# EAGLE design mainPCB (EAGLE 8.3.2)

## Sheet 1 of 2: RPi/ADC
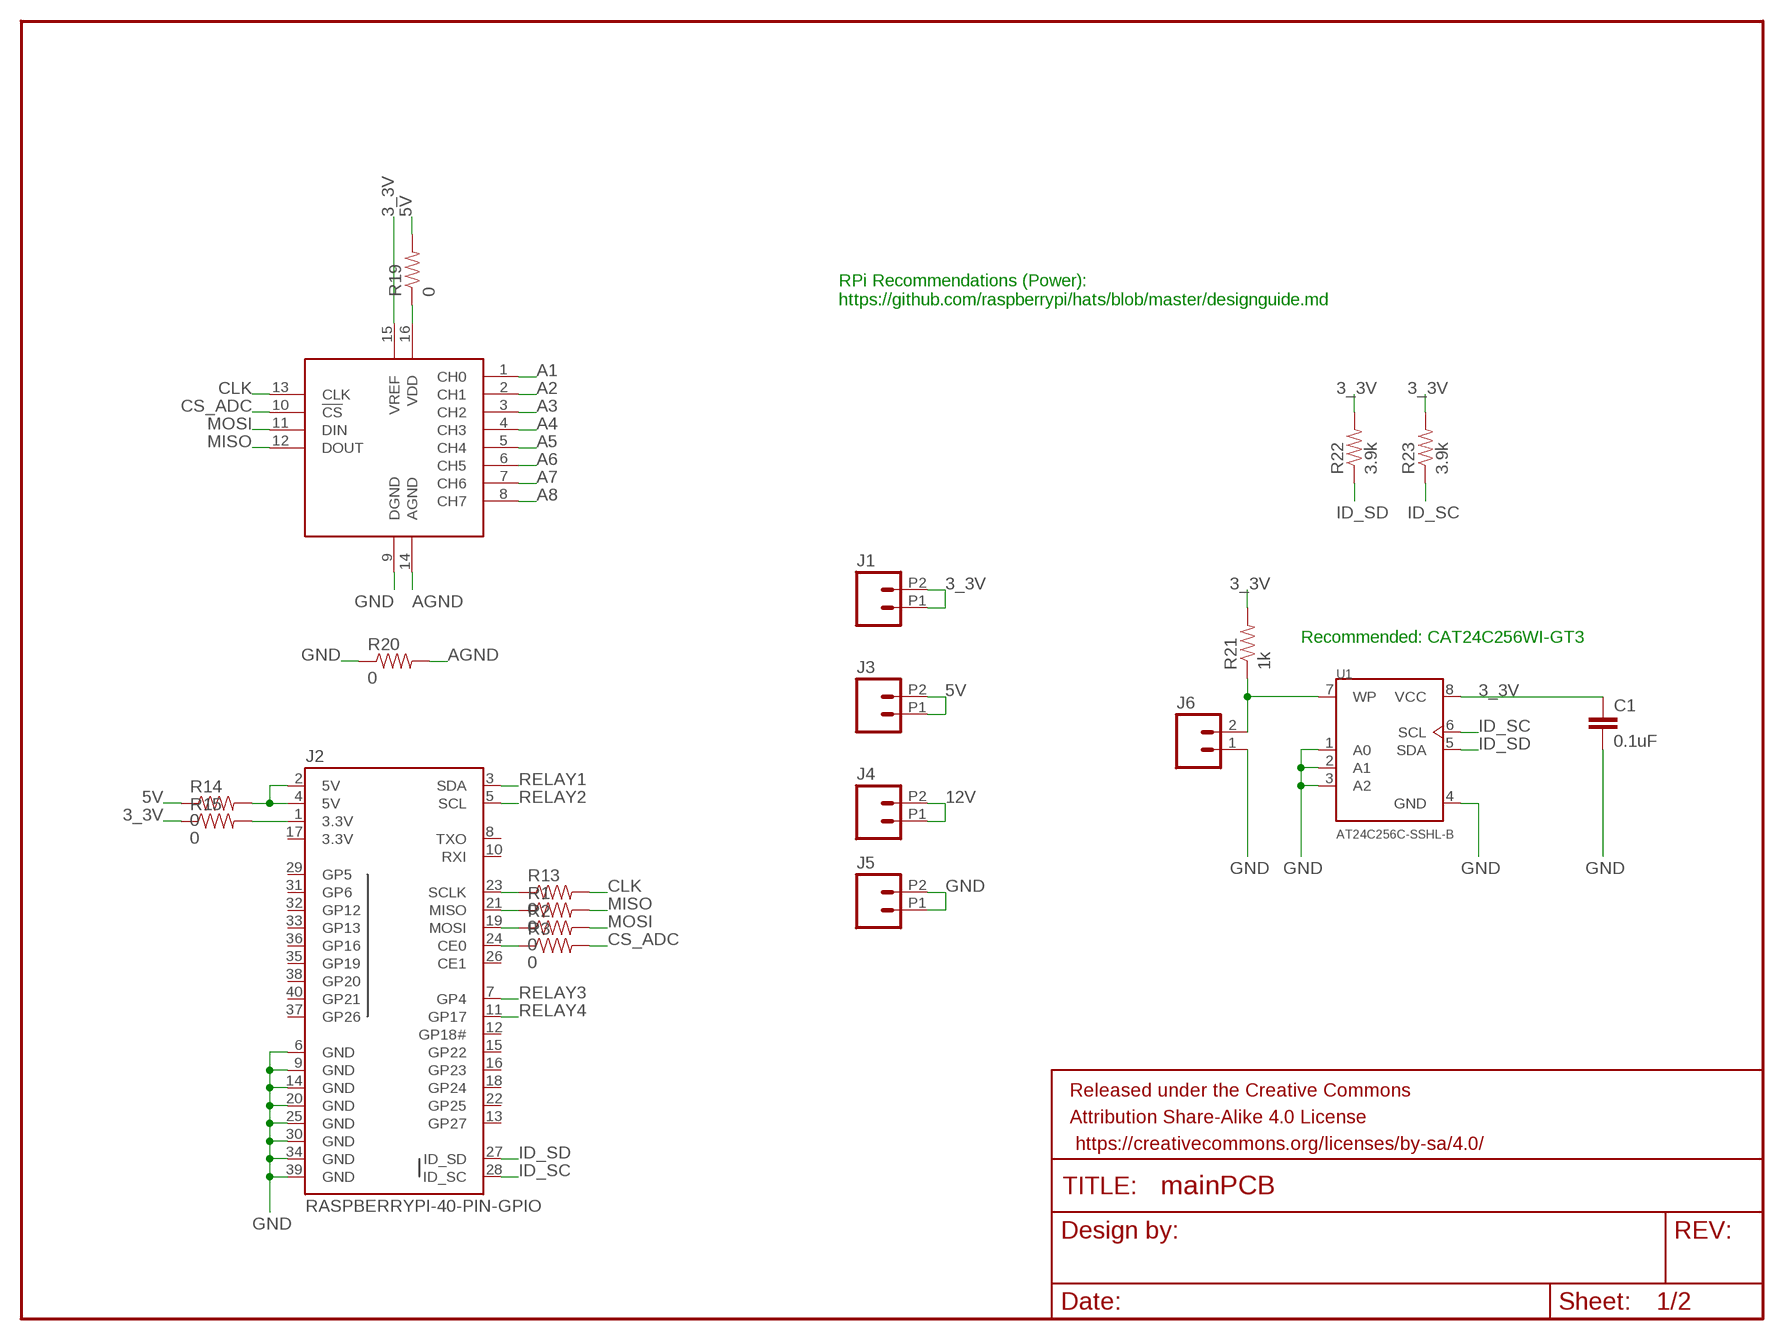
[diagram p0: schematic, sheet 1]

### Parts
C1  0.1uF  0.1UF-25V(+80/-20%)(0603)  [0603-CAP]
FRAME2  FRAME-LETTERNO_PACKAGE  [DUMMY]
J1  M022.54MM_SCREWTERM  [1X02_2.54_SCREWTERM]
J2  RASPBERRYPI-40-PIN-GPIO  [2X20-SHROUDED]
J3  M022.54MM_SCREWTERM  [1X02_2.54_SCREWTERM]
J4  M022.54MM_SCREWTERM  [1X02_2.54_SCREWTERM]
J5  M022.54MM_SCREWTERM  [1X02_2.54_SCREWTERM]
J6  M02PTH  [1X02]
R1  0  RESISTOR0603-RES  [0603-RES]
R2  0  RESISTOR0603-RES  [0603-RES]
R3  0  RESISTOR0603-RES  [0603-RES]
R13  0  RESISTOR0603-RES  [0603-RES]
R14  0  RESISTOR0603-RES  [0603-RES]
R15  0  RESISTOR0603-RES  [0603-RES]
R19  0  RESISTOR0603-RES  [0603-RES]
R20  0  RESISTOR0603-RES  [0603-RES]
R21  1k  RESISTOR0603-RES  [0603-RES]
R22  3.9k  RESISTOR0603-RES  [0603-RES]
R23  3.9k  RESISTOR0603-RES  [0603-RES]
U1  AT24C256C-SSHL-B  [SOIC127P600X175-8N]
U$1  MCP3208I/SL  [SO-16DW]

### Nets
3_3V: C1.1 J1.P1 J1.P2 R15.1 R21.2 R22.2 R23.2 U1.8(VCC) U$1.15(VREF)
5V: J3.P1 J3.P2 R14.1 R19.2 ; also sheet 2
12V: J4.P1 J4.P2 ; also sheet 2
A1: U$1.1(CH0) ; also sheet 2
A2: U$1.2(CH1) ; also sheet 2
A3: U$1.3(CH2) ; also sheet 2
A4: U$1.4(CH3) ; also sheet 2
A5: U$1.5(CH4)
A6: U$1.6(CH5)
A7: U$1.7(CH6)
A8: U$1.8(CH7)
AGND: R20.2 U$1.14(AGND)
CLK: R13.2 U$1.13(CLK)
CS_ADC: R3.2 U$1.10(!CS)
GND: C1.2 J2.6(GND) J2.9(GND) J2.14(GND) J2.20(GND) J2.25(GND) J2.30(GND) J2.34(GND) J2.39(GND) J5.P1 J5.P2 J6.1 R20.1 U1.1(A0) U1.2(A1) U1.3(A2) U1.4(GND) U$1.9(DGND) ; also sheet 2
ID_SC: J2.28(ID_SC) R23.1 U1.6(SCL)
ID_SD: J2.27(ID_SD) R22.1 U1.5(SDA)
MISO: R1.2 U$1.12(DOUT)
MOSI: R2.2 U$1.11(DIN)
N$17: J2.2(5V) J2.4(5V) R14.2
N$18: J2.1(3.3V) R15.2
N$19: J2.23(SCLK) R13.1
N$20: J2.21(MISO) R1.1
N$25: J2.19(MOSI) R2.1
N$26: J2.24(CE0) R3.1
N$27: R19.1 U$1.16(VDD)
RELAY1: J2.3(SDA) ; also sheet 2
RELAY2: J2.5(SCL) ; also sheet 2
RELAY3: J2.7(GP4) ; also sheet 2
RELAY4: J2.11(GP17) ; also sheet 2
WP: J6.2 R21.1 U1.7(WP)
Unconnected: J2.8(TXO) J2.10(RXI) J2.12(GP18#) J2.13(GP27) J2.15(GP22) J2.16(GP23) J2.18(GP24) J2.22(GP25) J2.26(CE1) J2.29(GP5) J2.31(GP6) J2.32(GP12) J2.33(GP13) J2.35(GP19) J2.36(GP16) J2.37(GP26) J2.38(GP20) J2.40(GP21)

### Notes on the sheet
- RPi Recommendations (Power):
  https://github.com/raspberrypi/hats/blob/master/designguide.md
- Recommended: CAT24C256WI-GT3

## Sheet 2 of 2: Relays 1-2
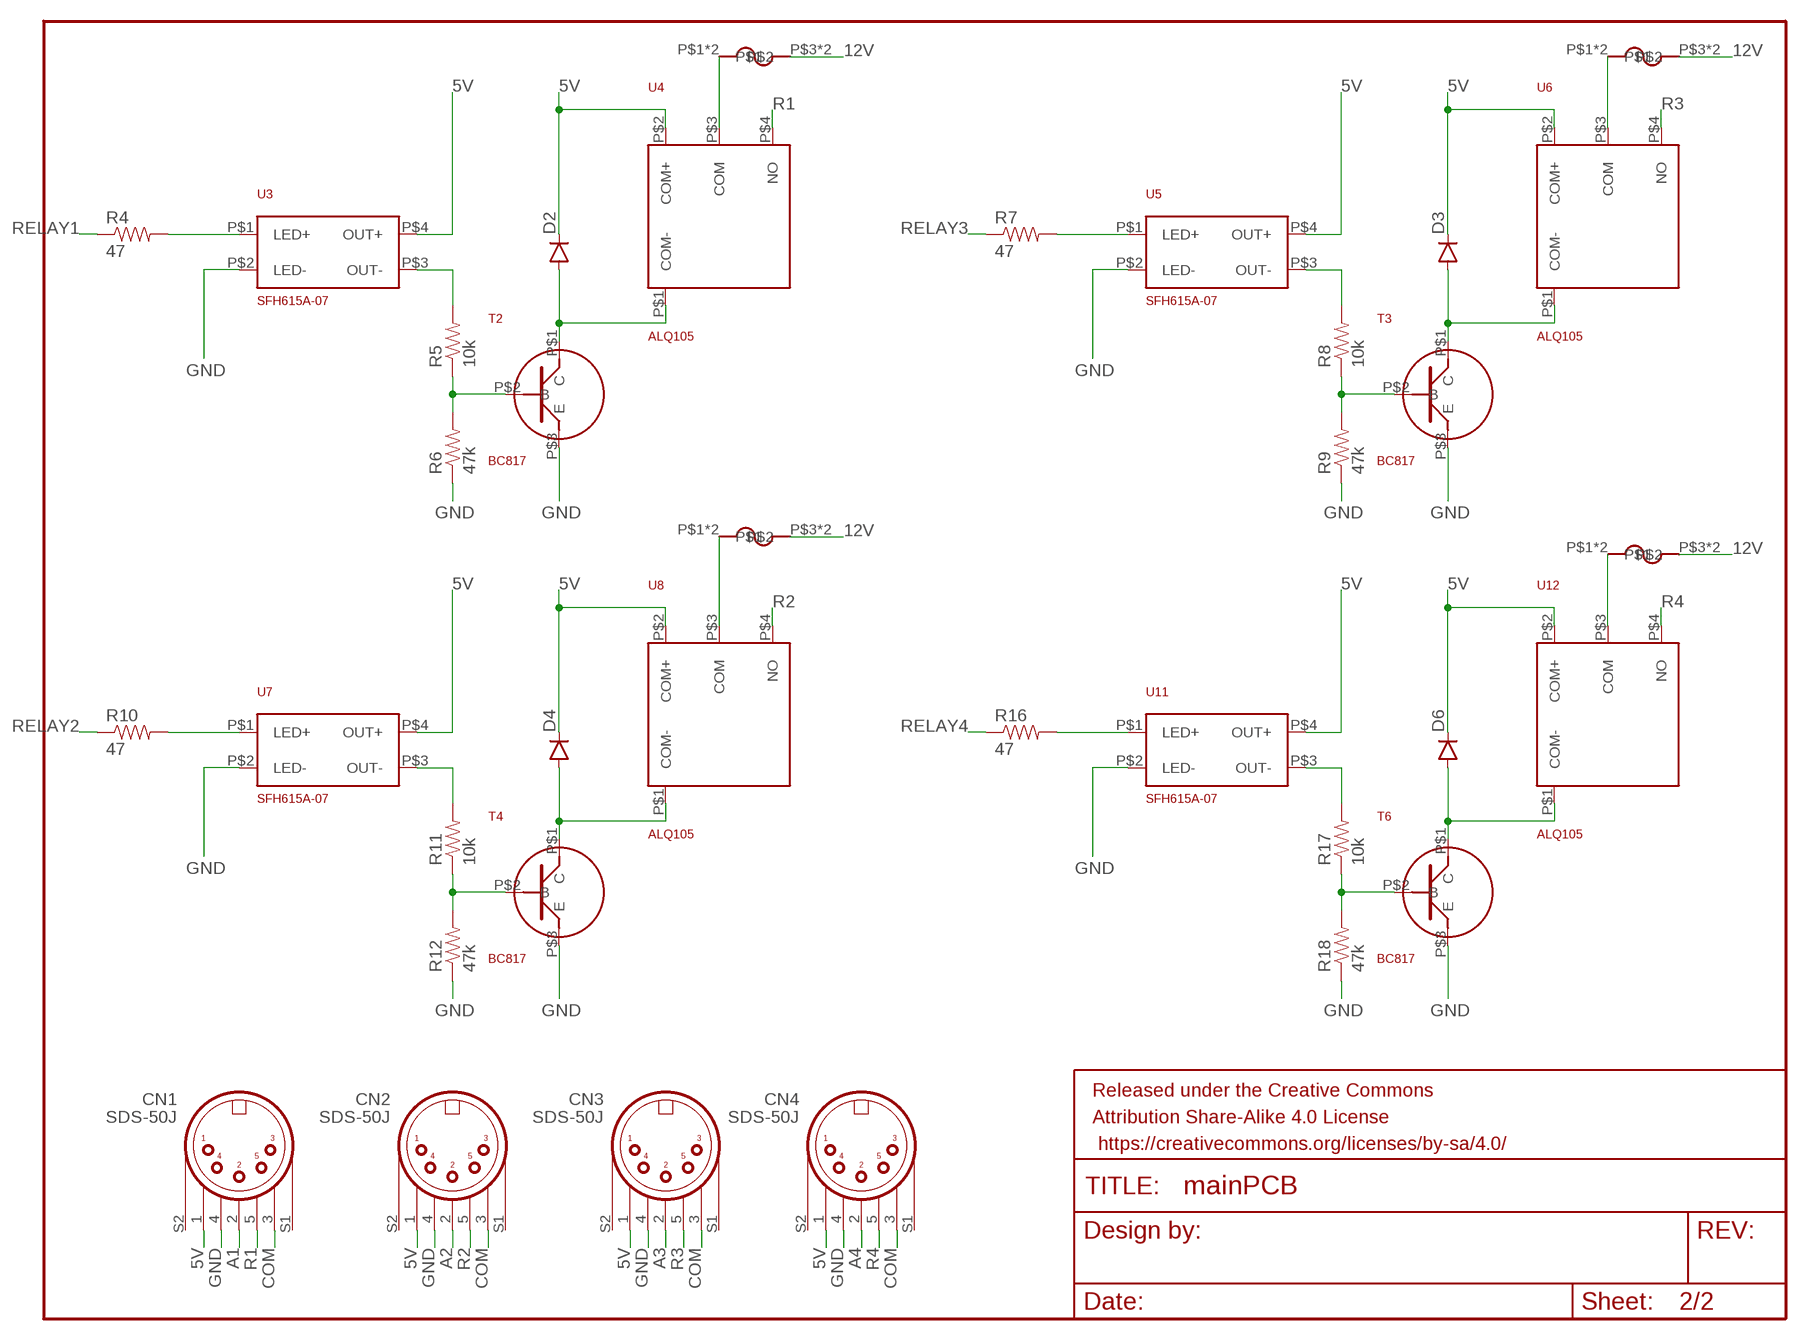
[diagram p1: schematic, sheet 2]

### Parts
CN1  SDS-50J  [SDS-50J]
CN2  SDS-50J  [SDS-50J]
CN3  SDS-50J  [SDS-50J]
CN4  SDS-50J  [SDS-50J]
D2  DIODESMA  [SMA-DIODE]
D3  DIODESMA  [SMA-DIODE]
D4  DIODESMA  [SMA-DIODE]
D6  DIODESMA  [SMA-DIODE]
F1  3544-2  [3544-2]
F2  3544-2  [3544-2]
F3  3544-2  [3544-2]
F4  3544-2  [3544-2]
FRAME1  FRAME-LETTERNO_PACKAGE  [DUMMY]
R4  47  RESISTOR0603-RES  [0603-RES]
R5  10k  RESISTOR0603-RES  [0603-RES]
R6  47k  RESISTOR0603-RES  [0603-RES]
R7  47  RESISTOR0603-RES  [0603-RES]
R8  10k  RESISTOR0603-RES  [0603-RES]
R9  47k  RESISTOR0603-RES  [0603-RES]
R10  47  RESISTOR0603-RES  [0603-RES]
R11  10k  RESISTOR0603-RES  [0603-RES]
R12  47k  RESISTOR0603-RES  [0603-RES]
R16  47  RESISTOR0603-RES  [0603-RES]
R17  10k  RESISTOR0603-RES  [0603-RES]
R18  47k  RESISTOR0603-RES  [0603-RES]
T2  BC817  [BC817]
T3  BC817  [BC817]
T4  BC817  [BC817]
T6  BC817  [BC817]
U3  SFH615A-07  [SFH615A-07]
U4  ALQ105  [ALQ105]
U5  SFH615A-07  [SFH615A-07]
U6  ALQ105  [ALQ105]
U7  SFH615A-07  [SFH615A-07]
U8  ALQ105  [ALQ105]
U11  SFH615A-07  [SFH615A-07]
U12  ALQ105  [ALQ105]

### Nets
5V: CN1.1 CN2.1 CN3.1 CN4.1 D2.C D3.C D4.C D6.C U3.P$4(OUT+) U4.P$2(COM+) U5.P$4(OUT+) U6.P$2(COM+) U7.P$4(OUT+) U8.P$2(COM+) U11.P$4(OUT+) U12.P$2(COM+) ; also sheet 1
12V: F1.P$3 F1.P$4 F2.P$3 F2.P$4 F3.P$3 F3.P$4 F4.P$3 F4.P$4 ; also sheet 1
A1: CN1.2 ; also sheet 1
A2: CN2.2 ; also sheet 1
A3: CN3.2 ; also sheet 1
A4: CN4.2 ; also sheet 1
COM: CN1.3 CN2.3 CN3.3 CN4.3
GND: CN1.4 CN2.4 CN3.4 CN4.4 R6.1 R9.1 R12.1 R18.1 T2.P$3(E) T3.P$3(E) T4.P$3(E) T6.P$3(E) U3.P$2(LED-) U5.P$2(LED-) U7.P$2(LED-) U11.P$2(LED-) ; also sheet 1
N$1: F1.P$1 F1.P$2 U4.P$3(COM)
N$2: F2.P$1 F2.P$2 U8.P$3(COM)
N$3: F4.P$1 F4.P$2 U12.P$3(COM)
N$4: F3.P$1 F3.P$2 U6.P$3(COM)
N$5: R4.2 U3.P$1(LED+)
N$6: R5.2 U3.P$3(OUT-)
N$7: R5.1 R6.2 T2.P$2(B)
N$8: D2.A T2.P$1(C) U4.P$1(COM-)
N$9: R7.2 U5.P$1(LED+)
N$10: R8.2 U5.P$3(OUT-)
N$11: R8.1 R9.2 T3.P$2(B)
N$12: D3.A T3.P$1(C) U6.P$1(COM-)
N$13: R10.2 U7.P$1(LED+)
N$14: R11.2 U7.P$3(OUT-)
N$15: R11.1 R12.2 T4.P$2(B)
N$16: D4.A T4.P$1(C) U8.P$1(COM-)
N$21: R16.2 U11.P$1(LED+)
N$22: R17.2 U11.P$3(OUT-)
N$23: R17.1 R18.2 T6.P$2(B)
N$24: D6.A T6.P$1(C) U12.P$1(COM-)
R1: CN1.5 U4.P$4(NO)
R2: CN2.5 U8.P$4(NO)
R3: CN3.5 U6.P$4(NO)
R4: CN4.5 U12.P$4(NO)
RELAY1: R4.1 ; also sheet 1
RELAY2: R10.1 ; also sheet 1
RELAY3: R7.1 ; also sheet 1
RELAY4: R16.1 ; also sheet 1
Unconnected: CN1.S1 CN1.S2 CN2.S1 CN2.S2 CN3.S1 CN3.S2 CN4.S1 CN4.S2

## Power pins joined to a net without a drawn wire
3.3V: J2.17(3.3V)

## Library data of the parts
C1 = SparkFun-Capacitors:0.1UF-25V(+80/-20%)(0603): CAP-00810; PROD_ID: CAP-00810
CN1-CN4 = SDS-50J:SDS-50J: DIN 5-Pin - Circular; AVAILABILITY: Good; DESCRIPTION: 5 Pin%2C Right-Angle Receptacle%2C 180%C2%B0; MF: CUI; MP: SDS-50J; PACKAGE: None; PRICE: 0.77 USD
D2-D4 D6 = SparkFun-DiscreteSemi:DIODE: Diode
F1-F4 = lib:3544-2: Keystone Electronics Fuse Holder - 3544-2
FRAME1 FRAME2 = SparkFun-Aesthetics:FRAME-LETTER: Schematic Frame; DESIGNER: Nobody; VERSION: v01
J1 J3-J6 = SparkFun-Connectors:M02: Standard 2-pin 0.1" header. Use with
J2 = SparkFun-Boards:RASPBERRYPI-40-PIN-GPIO: Second Generation Raspberry Pi GPIO Header 2x20 pin connector, as found on B, B+, A+ models.
R1-R23 = SparkFun-Passives:RESISTOR: Resistor
T2-T4 T6 = lib:BC817: NPN Transistor BC817 Data sheet
U1 = AT24C256C-SSHL-B:AT24C256C-SSHL-B: EEPROM Serial-2Wire 256K-bit 32K x 8 1.8V/2.5V/3.3V/5V 8-Pin SOIC Bulk; DESCRIPTION: EEPROM Serial-2Wire 256K-bit 32K x 8 1.8V/2.5V/3.3V/5V 8-Pin SOIC Bulk; DIGI-KEY_PART_NUMBER: AT24C256C-SSHL-B-ND; DIGI-KEY_PURCHASE_URL: https://www.digikey.com/product-detail/en/microchip-technology/AT24C256C-SSHL-B/AT24C256C-SSHL-B-ND/2271121?WT.z_cid=ref_snapeda; MF: Atmel; MP: AT24C256C-SSHL-B; PACKAGE: SOIC-8 Atmel
U3 U5 U7 U11 = lib:SFH615A-07: Vishay Optocoupler SFH615A-007 Data sheet
U4 U6 U8 U12 = lib:ALQ105: ALQ105 Solenoid Data sheet
U$1 = adcLib:MCP3208: Microchip MCP3208 8-bit ADC

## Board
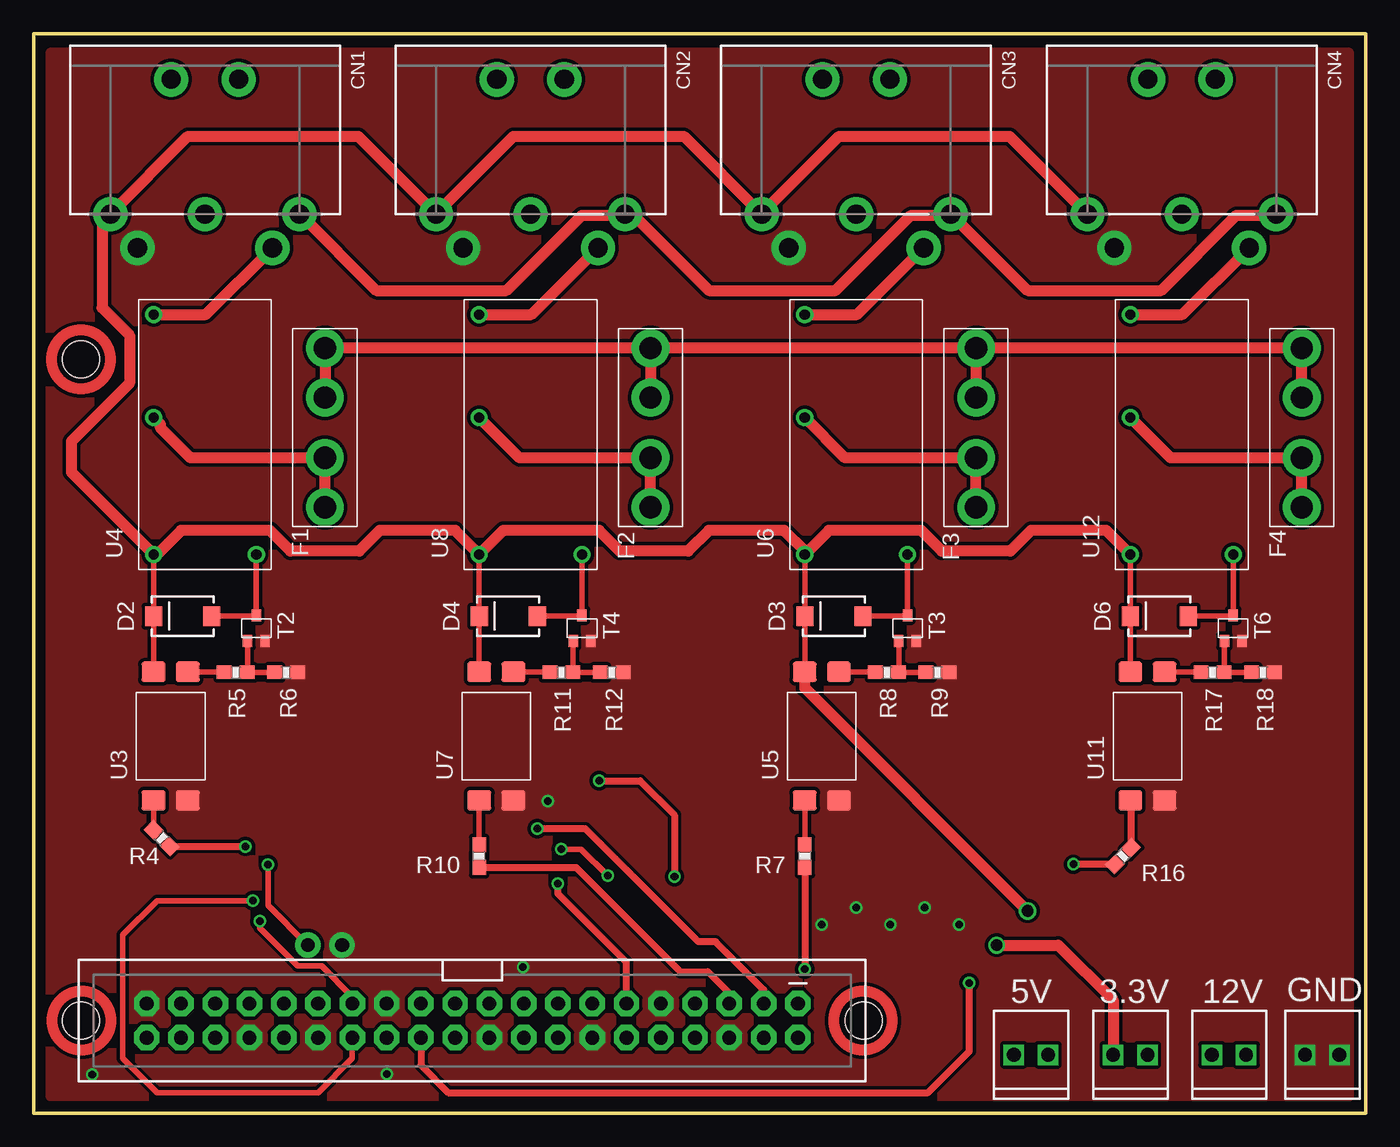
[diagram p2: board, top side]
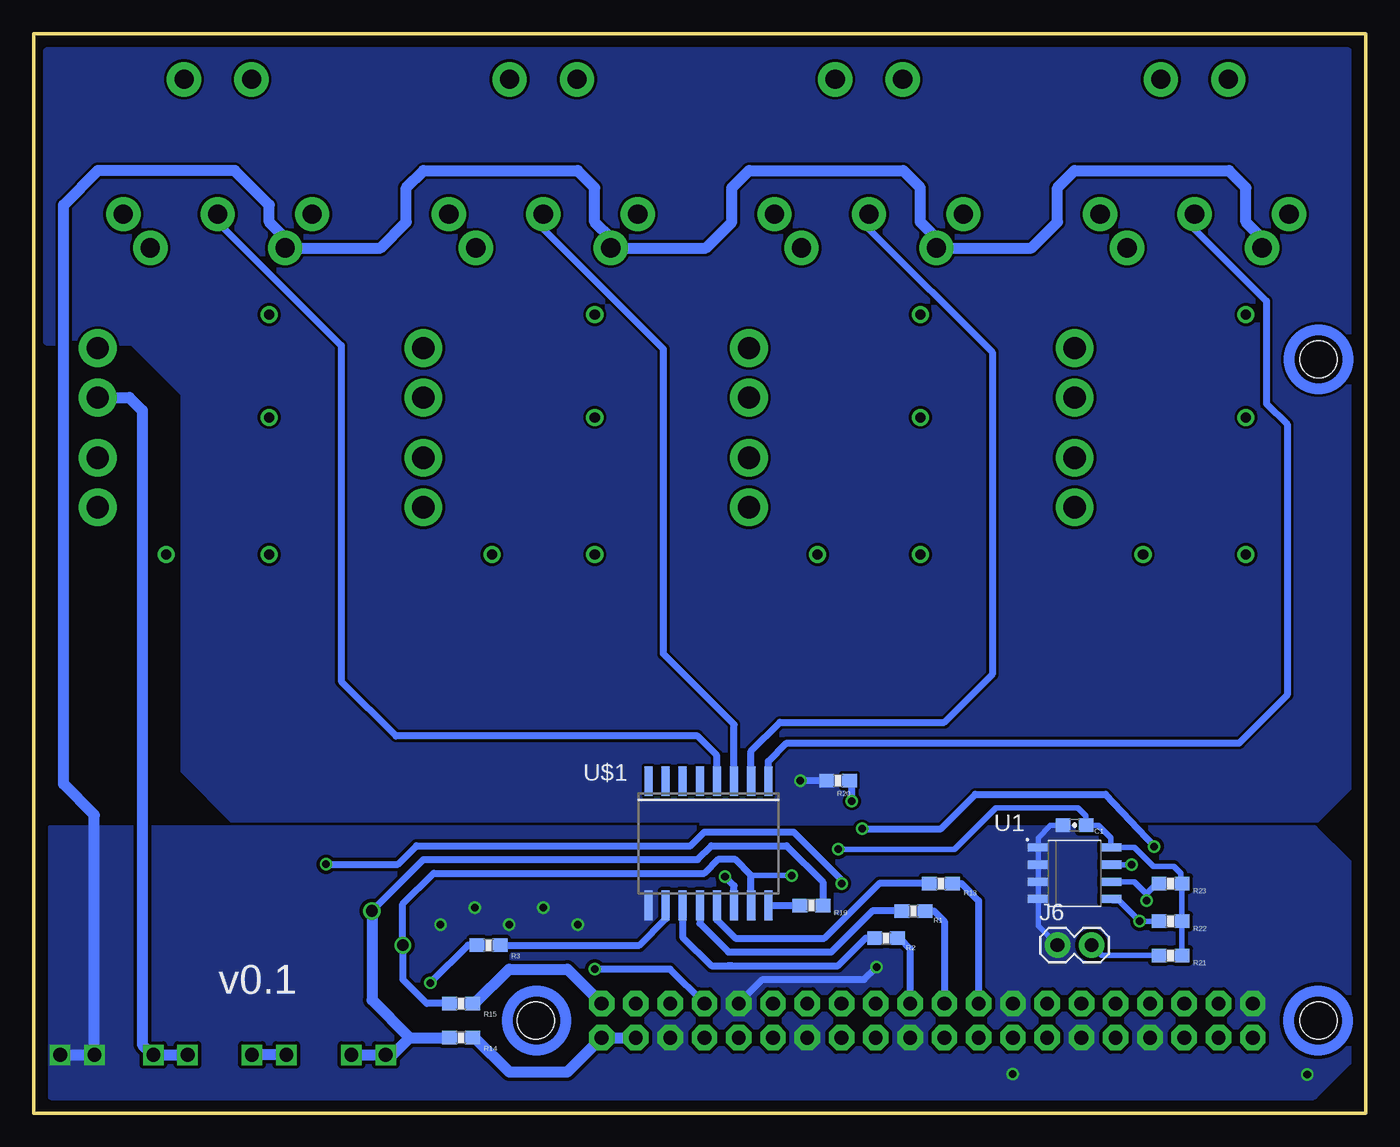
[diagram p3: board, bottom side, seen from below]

Size 98.72 x 80 mm. Coordinates in mm from the lower left corner, seen from the top.
Outline: 0,0 98.72,0 98.72,80 0,80 0,0
Copper layers (1*16): Top 0.0356mm / dielectric 1.5011mm / Bottom 0.0356mm
Design rules "oshpark-2layer": minimum track width 6mil, minimum drill 13mil, track to track 6mil, track to pad 6mil, pad to pad 6mil, via to via 6mil, smd to smd 6mil, copper to edge 15mil, drill to drill 6mil, minimum pad ring 7mil, minimum via ring 7mil, stop-mask expansion 2.5mil, vias tented up to drill 0mil, thermal gap 10mil
Holes 2.75 mm at 3.5,6.86 61.5,6.86 3.5,55.86

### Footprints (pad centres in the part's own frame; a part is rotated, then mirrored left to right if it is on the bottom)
0603-CAP = smd 1.1 x 1: 1 -0.85,0; 2 0.85,0
SDS-50J = drill 1.422 pad 2.54: 1 7,4.5; 2 0,4.5; 3 -7,4.5; 4 5,7; 5 -5,7; S1 -2.5,-5.5; S2 2.5,-5.5
SMA-DIODE = smd 1.27 x 1.47: A -2.15,0; C 2.15,0
3544-2 = drill 1.65 pad 2.8: P$1 -5.895,0; P$2 -2.235,0; P$3 2.235,0; P$4 5.895,0
1X02_2.54_SCREWTERM = drill 1.016 square: P1 2.54,0; P2 0,0
2X20-SHROUDED = drill 1.016 pad 1.88 octagon: 1 -1.27,24.13; 2 1.27,24.13; 3 -1.27,21.59; 4 1.27,21.59; 5 -1.27,19.05; 6 1.27,19.05; 7 -1.27,16.51; 8 1.27,16.51; 9 -1.27,13.97; 10 1.27,13.97; 11 -1.27,11.43; 12 1.27,11.43; 13 -1.27,8.89; 14 1.27,8.89; 15 -1.27,6.35; 16 1.27,6.35; 17 -1.27,3.81; 18 1.27,3.81; 19 -1.27,1.27; 20 1.27,1.27; 21 -1.27,-1.27; 22 1.27,-1.27; 23 -1.27,-3.81; 24 1.27,-3.81; 25 -1.27,-6.35; 26 1.27,-6.35; 27 -1.27,-8.89; 28 1.27,-8.89; 29 -1.27,-11.43; 30 1.27,-11.43; 31 -1.27,-13.97; 32 1.27,-13.97; 33 -1.27,-16.51; 34 1.27,-16.51; 35 -1.27,-19.05; 36 1.27,-19.05; 37 -1.27,-21.59; 38 1.27,-21.59; 39 -1.27,-24.13; 40 1.27,-24.13
1X02 = drill 1.016 pad 1.88: 1 0,0; 2 2.54,0
0603-RES = smd 1.1 x 1: 1 -0.85,0; 2 0.85,0
BC817 = smd 0.7 x 0.9: P$1 0,0.95; P$2 -0.65,-0.95; P$3 0.65,-0.95
SOIC127P600X175-8N = smd 1.55 x 0.6: 1 -2.7,1.905; 2 -2.7,0.635; 3 -2.7,-0.635; 4 -2.7,-1.905; 5 2.7,-1.905; 6 2.7,-0.635; 7 2.7,0.635; 8 2.7,1.905
SFH615A-07 = smd 1.52 x 1.78: P$1 -4.765,1.27; P$2 -4.765,-1.27; P$3 4.765,-1.27; P$4 4.765,1.27
ALQ105 = drill 0.75 pad 1.27: P$1 0,0; P$2 0,7.62; P$3 10.16,7.62; P$4 17.78,7.62
SO-16DW = smd 0.6 x 2.2: 1 -4.445,-4.6; 2 -3.175,-4.6; 3 -1.905,-4.6; 4 -0.635,-4.6; 5 0.635,-4.6; 6 1.905,-4.6; 7 3.175,-4.6; 8 4.445,-4.6; 9 4.445,4.6; 10 3.175,4.6; 11 1.905,4.6; 12 0.635,4.6; 13 -0.635,4.6; 14 -1.905,4.6; 15 -3.175,4.6; 16 -4.445,4.6

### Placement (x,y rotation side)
C1  21.58,21.34 180 bottom
CN1  12.69,71.12 180 top
CN2  36.82,71.12 180 top
CN3  60.95,71.12 180 top
CN4  85.08,71.12 180 top
D2  11.04,36.83 180 top
D3  59.3,36.83 180 top
D4  35.17,36.83 180 top
D6  83.43,36.83 180 top
F1  21.58,50.8 90 top
F2  45.71,50.8 90 top
F3  69.84,50.8 90 top
F4  93.97,50.8 90 top
FRAME1  97.4,11.51 0 top
FRAME2  97.4,13.36 0 top
J1  82.54,4.32 180 top
J2  32.5,6.86 270 top
J3  75.17,4.32 180 top
J4  89.86,4.32 180 top
J5  96.76,4.32 180 top
J6  22.85,12.45 0 bottom
R1  33.52,14.99 180 bottom
R2  35.55,12.95 180 bottom
R3  65.01,12.45 0 bottom
R4  9.49,20.37 135 top
R5  14.98,32.66 180 top
R6  18.71,32.66 180 top
R7  57.14,19.05 90 top
R8  63.24,32.66 180 top
R9  66.97,32.66 180 top
R10  33.01,19.05 90 top
R11  39.11,32.66 180 top
R12  42.84,32.66 180 top
R13  31.49,17.02 180 bottom
R14  67.05,5.59 0 bottom
R15  67.05,8.13 0 bottom
R16  80.71,19.05 45 top
R17  87.37,32.66 180 top
R18  91.1,32.66 180 top
R19  41.09,15.39 0 bottom
R20  39.11,24.64 180 bottom
R21  14.47,11.68 0 bottom
R22  14.47,14.22 0 bottom
R23  14.47,17.02 0 bottom
T2  16.5,35.94 0 top
T3  64.76,35.94 0 top
T4  40.63,35.94 0 top
T6  88.89,35.94 0 top
U1  21.58,17.78 0 bottom
U3  10.15,27.94 90 top
U4  16.5,41.4 90 top
U5  58.41,27.94 90 top
U6  64.76,41.4 90 top
U7  34.28,27.94 90 top
U8  40.63,41.4 90 top
U11  82.54,27.94 90 top
U12  88.89,41.4 90 top
U$1  48.72,20 180 bottom

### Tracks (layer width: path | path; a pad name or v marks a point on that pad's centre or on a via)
3_3V  (via drill 0.56, 0.84)
  Top 0.406: v42.53,17.6 40.58,19.56 v39.11,19.56
  Top 0.813: J1.P1 80,8.38 75.94,12.45 v71.36,12.45
  Bottom 0.406: R21.2 R22.2 R23.2 13.71,17.11 13.71,17.78 14.21,18.29 15.74,18.29 17.13,19.68 U1.8 18.88,20.41 19.8,21.34 C1.1 20.73,22.01 21.33,22.61 27.42,22.61 30.47,19.56 v39.11,19.56 | v42.53,17.6 45.53,17.6 45.55,17.61
  Bottom 0.508: R15.1 69.59,8.13 71.36,9.91 v71.36,12.45 71.36,15.49 69.08,17.78 49.01,17.78 48,18.8 46.73,18.8 45.55,17.61 U$1.15
  Bottom 0.813: J1.P1 J1.P2
5V  (via drill 0.86)
  Top 0.406: U3.P$4 D2.C U4.P$2 | U7.P$4 D4.C U8.P$2 | U5.P$4 D3.C U6.P$2 | U11.P$4 D6.C U12.P$2
  Top 0.813: CN4.1 72.31,72.39 59.68,72.39 53.95,66.66 CN3.1 48.18,72.39 35.55,72.39 29.82,66.66 CN2.1 24.05,72.39 11.42,72.39 5.69,66.66 CN1.1 5.65,66.62 5.07,66.04 5.07,59.69 7.1,57.66 7.1,54.1 2.78,49.78 2.78,47.5 U4.P$2 9.13,41.4 10.91,43.18 17.52,43.18 19.04,41.66 24.12,41.66 25.64,43.18 31.23,43.18 U8.P$2 34.79,43.18 41.9,43.18 43.42,41.66 48.5,41.66 50.03,43.18 55.62,43.18 57.14,41.66 U6.P$2 58.92,43.18 65.78,43.18 67.3,41.66 72.38,41.66 73.9,43.18 79.49,43.18 U12.P$2 | v73.65,14.99 57.14,31.5 U5.P$4
  Bottom 0.508: R19.2 40.24,17.13 42.92,19.81 48.5,19.81 49.52,18.8 69.84,18.8 v73.65,14.99
  Bottom 0.813: 70.86,5.59 R14.1 | 70.86,5.59 73.65,8.38 v73.65,14.99 | J3.P2 J3.P1 72.13,4.32 70.86,5.59
12V
  Top 0.813: 69.84,56.39 F3.P$3 | 69.84,56.39 F3.P$4 46.02,56.7 45.71,56.39 | F1.P$3 F1.P$4 F2.P$4 45.71,56.39 | 45.71,56.39 F2.P$3 | F4.P$3 F4.P$4 70.15,56.7 69.84,56.39
  Bottom 0.813: J4.P1 J4.P2 89.91,4.37 89.91,4.32 90.67,5.08 90.67,52.07 91.63,53.03 F4.P$3
A1
  Bottom 0.508: CN1.2 12.69,65.53 7.36,60.2 7.36,52.58 5.83,51.05 5.83,30.99 9.39,27.43 42.92,27.43 44.27,26.07 U$1.1
A2
  Bottom 0.508: CN2.2 36.82,65.53 27.68,56.39 27.68,32.51 31.23,28.96 43.42,28.96 45.55,26.84 U$1.2
A3
  Bottom 0.508: CN3.2 60.95,65.53 52.06,56.64 52.06,34.04 46.81,28.79 U$1.3
A4
  Bottom 0.508: 85.08,66.04 75.94,56.9 75.94,32 71.87,27.94 49.52,27.94 48.09,26.5 U$1.4
  Bottom 0.813: CN4.2 85.08,66.04
AGND  (via drill 0.56)
  Top 0.508: v41.9,24.64 44.95,24.64 47.49,22.1 v47.49,17.53
  Bottom 0.508: U$1.14 46.81,16.85 v47.49,17.53 | R20.2 v41.9,24.64
  pour Bottom (isolate 0.203, rank 3, no thermals): 1.29,78.74 97.78,78.74 97.78,57.15 91.43,57.15 87.62,53.34 87.62,25.4 83.81,21.59 3.8,21.59 1.29,24.1 1.29,24.13
CLK
  Bottom 0.508: R13.2 36.06,17.02 40.12,12.95 46.73,12.95 48.09,14.31 U$1.13
COM
  Top 0.813: CN1.3 19.73,66.62 25.39,60.96 35.04,60.96 40.63,66.55 43.89,66.55 | 43.89,66.55 44.44,66.55 50.03,60.96 59.43,60.96 65.01,66.55 67.88,66.55 CN3.3 67.99,66.62 73.65,60.96 83.56,60.96 89.14,66.55 92.01,66.55 CN4.3 | 43.89,66.55 CN2.3
CS_ADC
  Bottom 0.508: U$1.10 51.89,14.39 53.84,12.45 R3.2
GND  (via drill 0.56)
  Bottom 0.406: C1.2 23.36,21.34 24.28,20.41 U1.1 U1.2 U1.3 U1.4 24.28,13.88 J6.1
  Bottom 0.508: v36.26,10.82 37.18,9.91 44.69,9.91 J2.9 | v38.09,23.11 38.09,24.47 R20.1
  Bottom 0.813: CN1.4 7.69,64.85 8.88,66.04 8.88,68.58 10.15,69.85 21.58,69.85 22.85,68.58 22.85,66.04 24.77,64.12 CN2.4 31.82,64.85 33.01,66.04 33.01,68.58 34.28,69.85 45.71,69.85 46.98,68.58 46.98,66.04 48.9,64.12 CN3.4 55.95,64.85 57.14,66.04 57.14,68.58 58.41,69.85 69.84,69.85 71.11,68.58 71.11,66.04 73.03,64.12 CN4.4 80.08,64.85 81.27,66.04 81.27,67.31 83.81,69.85 93.97,69.85 96.51,67.31 96.51,24.38 94.22,22.1 J5.P1 J5.P2
  other vias: 58.41,13.97 60.95,15.24 63.49,13.97 66.03,15.24 68.57,13.97 26.18,2.9 4.33,2.87
  pour Top (isolate 0.254, no thermals): 97.42,78.59 97.42,1.27 1.29,1.27 1.29,78.59
  pour Bottom (isolate 0.254, no thermals): 97.42,1.22 3.9,1.22 3.8,1.27 1.29,3.78 1.29,18.57 3.8,21.08 97.4,21.09 97.42,21.11
ID_SC  (via drill 0.56)
  Top 0.406: J2.28 23.61,4.06 21.07,1.52 9.13,1.52 6.59,4.06 6.59,13.21 9.13,15.75 v16.25,15.75
  Bottom 0.406: 15.4,17.1 15.45,17.14 | 15.4,17.1 R23.1 | 16.25,16.26 v16.25,15.75 | 16.25,16.26 15.4,17.1 | U1.6 17.13,17.14 16.25,16.26
ID_SD  (via drill 0.56)
  Top 0.406: J2.27 23.61,8.64 21.33,10.92 19.55,10.92 16.75,13.72 v16.75,14.22
  Bottom 0.406: U1.5 18.75,15.75 18.28,15.75 v16.75,14.22 R22.1
MISO
  Bottom 0.508: R1.2 36.57,14.99 39.61,11.94 47.23,11.94 49.35,14.06 U$1.12
MOSI
  Bottom 0.508: R2.2 37.07,12.95 39.11,10.92 46.98,10.92 | 46.98,10.92 47.23,10.92 | U$1.11 50.62,13.04 48.5,10.92 46.98,10.92
N$1
  Top 0.813: F1.P$1 F1.P$2 11.62,48.56 9.39,50.8 9.39,51.05 U4.P$3
N$2
  Top 0.813: F2.P$1 F2.P$2 36.01,48.56 U8.P$3
N$3
  Top 0.813: F4.P$1 F4.P$2 84.27,48.56 U12.P$3
N$4
  Top 0.813: F3.P$1 70.04,44.7 70.35,44.7 69.84,45.21 F3.P$2 60.14,48.56 U6.P$3
N$5
  Top 0.406: R4.2 U3.P$1
N$6
  Top 0.406: U3.P$3 14.09,32.7 R5.2
N$7
  Top 0.406: 15.85,32.72 T2.P$2 | 15.85,32.72 15.85,32.69 R5.1 | R6.2 15.9,32.66 15.85,32.72
N$8
  Top 0.406: D2.A 16.44,36.83 T2.P$1 U4.P$1
N$9
  Top 0.406: R7.2 U5.P$1
N$10
  Top 0.406: U5.P$3 62.34,32.7 R8.2
N$11
  Top 0.406: 64.11,32.72 T3.P$2 | 64.11,32.72 64.11,32.69 R8.1 | R9.2 64.16,32.66 64.11,32.72
N$12
  Top 0.406: D3.A 64.7,36.83 T3.P$1 U6.P$1
N$13
  Top 0.406: R10.2 U7.P$1
N$14
  Top 0.406: U7.P$3 38.21,32.7 R11.2
N$15
  Top 0.406: 39.98,32.72 T4.P$2 | 39.98,32.72 39.98,32.69 R11.1 | R12.2 40.03,32.66 39.98,32.72
N$16
  Top 0.406: D4.A 40.57,36.83 T4.P$1 U8.P$1
N$17
  Bottom 0.813: R14.2 66.03,5.59 63.49,3.05 59.17,3.05 J2.2 J2.4
N$18
  Bottom 0.813: R15.2 66.03,8.13 63.49,10.67 59.17,10.67 J2.1
N$19
  Bottom 0.508: R13.1 29.96,17.02 28.69,15.75 J2.23
N$20
  Bottom 0.508: R1.1 31.99,14.99 31.23,14.22 J2.21
N$21
  Top 0.508: U11.P$1 81.31,23.13 R16.2
N$22
  Top 0.406: U11.P$3 86.47,32.7 R17.2
N$23
  Top 0.406: 88.24,32.72 T6.P$2 | 88.24,32.72 88.24,32.69 R17.1 | R18.2 88.29,32.66 88.24,32.72
N$24
  Top 0.406: D6.A 88.83,36.83 T6.P$1 U12.P$1
N$25
  Bottom 0.508: R2.1 34.53,12.95 33.77,12.19 J2.19
N$26  (via drill 0.56)
  Top 0.508: J2.24 28.69,3.56 30.72,1.52 66.28,1.52 69.33,4.57 v69.33,9.65
  Bottom 0.508: R3.1 66.54,12.45 v69.33,9.65
N$27
  Bottom 0.508: U$1.16 R19.1
R1
  Top 0.813: U4.P$4 12.75,59.18 CN1.5
R2
  Top 0.813: U8.P$4 36.88,59.18 CN2.5
R3
  Top 0.813: U6.P$4 61.01,59.18 CN3.5
R4
  Top 0.813: U12.P$4 85.14,59.18 CN4.5
RELAY1  (via drill 0.56)
  Top 0.508: J2.3 54.09,9.14 50.54,12.7 49.27,12.7 40.88,21.08 v37.33,21.08 | R4.1 v15.69,19.76
  Bottom 0.508: v37.33,21.08 31.49,21.08 28.95,23.62 19.29,23.62 v15.69,19.76
RELAY2
  Top 0.508: J2.5 51.55,8.89 49.97,10.47 47.94,10.47 40.21,18.2 R10.1
RELAY3  (via drill 0.56)
  Top 0.508: R7.1 v57.14,10.67
  Bottom 0.508: J2.7 51.55,10.67 v57.14,10.67
RELAY4  (via drill 0.56)
  Top 0.508: J2.11 43.93,11.18 38.85,16.26 v38.85,17.02 | R16.1 v77.05,18.44
  Bottom 0.508: v77.05,18.44 71.72,18.44 70.35,19.81 50.03,19.81 49.01,20.83 42.41,20.83 38.85,17.27 v38.85,17.02
WP  (via drill 0.56)
  Top 0.406: v17.36,18.41 17.36,15.39 J6.2
  Bottom 0.406: R21.1 19.55,11.68 J6.2 | U1.7 v17.36,18.41
(copper drawn outside any net)
  shapes: Bottom circle x3, Top circle x3

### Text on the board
tPlace: 5V | 3.3V | 12V | GND
bNames: v0.1

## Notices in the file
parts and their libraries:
SparkFun-Passives: Licensing: Creative Commons ShareAlike 4.0 International - https://creativecommons.org/licenses/by-sa/4.0
SparkFun-Aesthetics: Released under the Creative Commons Attribution Share-Alike 4.0 License
SparkFun-Aesthetics: https://creativecommons.org/licenses/by-sa/4.0
